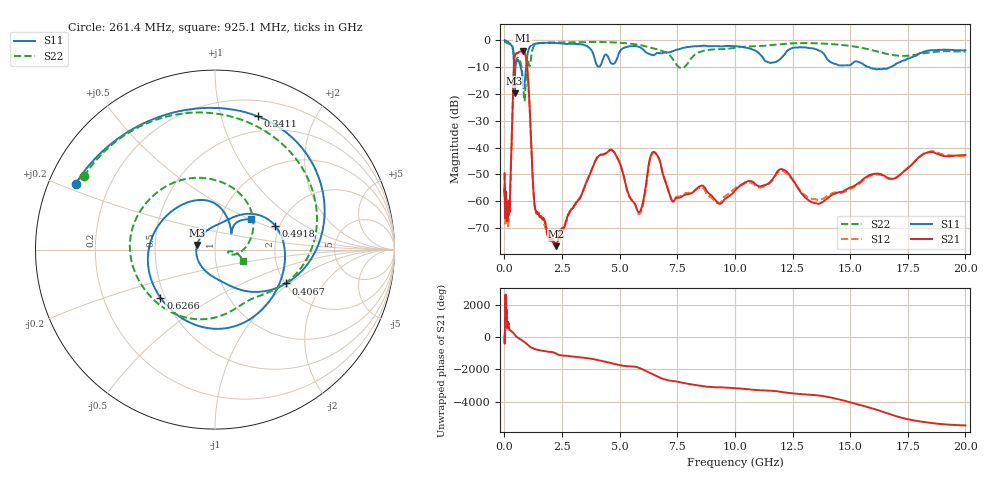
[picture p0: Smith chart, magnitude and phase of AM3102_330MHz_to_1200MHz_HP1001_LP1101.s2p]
! Date/Time: Tue, Sep 11, 2018 5:18 PM
! Network Analyzer: Agilent Technologies E8362B Rev: A.07.50.63
! Sweep from 0.010 to 20.000 GHz, 1601 Points, Sweep Type: LOG
! Power Supply: 4.949 V, 0.001 A
# Hz S DB R 50
!freq MagS11 AngS11 MagS21 AngS21 MagS12 AngS12 MagS22 AngS22
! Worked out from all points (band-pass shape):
!   1601 points, 10 MHz to 20 GHz, reference 50 ohm
!   highest |S21| = -3.80 dB at 798.4 MHz (marker M1); lowest = -76.7 dB at 2.26 GHz (marker M2)
!   |S21| within 3 dB of the highest: 431.7 MHz to 944.8 MHz (513.2 MHz wide, 74.6 % of centre)
!   lowest |S11| = -19.7 dB at 443 MHz (marker M3), VSWR 1.23, Z = 40.8 + j2.16 ohm
!   |S11| at or under -10 dB: 415.9 MHz to 479.2 MHz (63.26 MHz wide, 14.1 % of centre); 706.9 MHz to 942 MHz (235.1 MHz wide, 28.5 % of centre); 15.84 GHz to 16.73 GHz (894 MHz wide, 5.49 % of centre)
!   |S22| runs from -22.7 to -0.2 dB; largest |S21 - S12| = 0.0096
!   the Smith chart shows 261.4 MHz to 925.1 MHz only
!   S11 on the Smith chart (normalised r, x): 261.4 MHz: 0.08, +0.22; 341.1 MHz: 0.35, +1.31; 406.7 MHz: 2.02, -0.94; 491.8 MHz: 1.90, +0.57; 626.6 MHz: 0.47, -0.30; 925.1 MHz: 1.40, +0.50
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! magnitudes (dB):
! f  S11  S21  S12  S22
! 10 MHz  0.0  -49.6  -49.5  -0.2
! 35.55 MHz  0.0  -62.9  -62.9  -0.5
! 126.4 MHz  -0.4  -66.5  -65.1  -1.0
! 261.4 MHz  -1.3  -53.2  -53.9  -1.6
! 341.1 MHz  -2.2  -29.9  -29.9  -2.5
! 406.7 MHz  -7.2  -10.8  -10.8  -5.9
! 443 MHz  -19.7  -5.9  -6.0  -9.3
! 447.2 MHz  -19.5  -5.7  -5.8  -9.4
! 491.8 MHz  -8.8  -5.0  -5.0  -7.9
! 626.6 MHz  -7.8  -4.3  -4.4  -6.8
! 798.4 MHz  -15.8  -3.8  -3.9  -14.1
! 925.1 MHz  -11.6  -5.8  -5.9  -15.4
! 1.296 GHz  -1.4  -60.1  -60.7  -2.0
! 1.59 GHz  -1.0  -66.0  -65.4  -0.9
! 2.26 GHz  -1.0  -76.7  -75.5  -0.7
! 4.5 GHz  -6.1  -41.4  -41.3  -0.6
! 5.652 GHz  -2.1  -60.8  -61.1  -1.4
! 6.518 GHz  -5.3  -41.7  -41.9  -3.0
! 7.41 GHz  -3.6  -59.2  -58.8  -8.3
! 12.03 GHz  -6.4  -48.0  -48.5  -1.4
! 13.55 GHz  -3.3  -60.8  -59.4  -1.1
! 20 GHz  -3.7  -42.7  -43.2  -4.2
